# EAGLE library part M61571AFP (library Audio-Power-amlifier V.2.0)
M61571AFP is a Digital power amplifier IC developed for home audio. M61571AFP can realize maximum Power 50W × 2ch(VD = 21V,THD = 10%, BTL) at 4 Ω load. It is possible to replace from the conventional analog amplifier system to the digital amplifier system easily. Refer to "http://www.renesas.com/en/network" for the latest and detailed information.
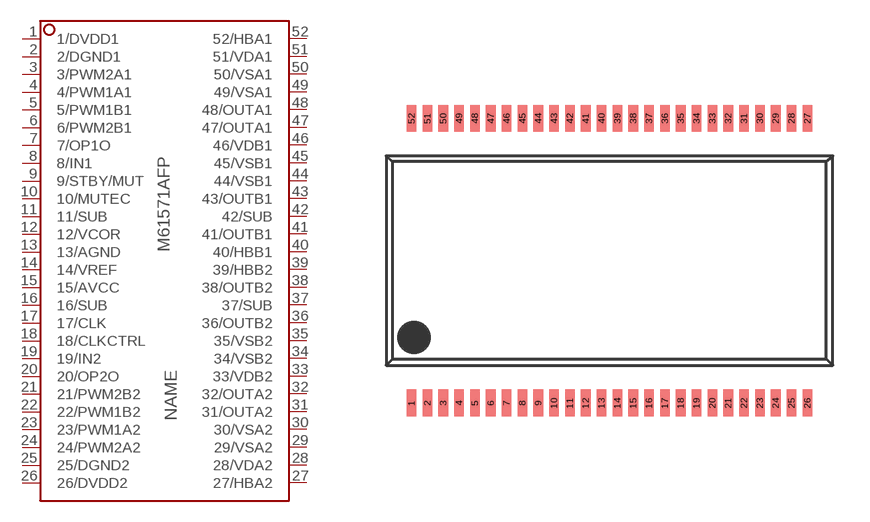
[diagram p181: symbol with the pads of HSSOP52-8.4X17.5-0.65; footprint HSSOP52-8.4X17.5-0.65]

Designator prefix IC

## M61571AFP  [HSSOP52-8.4X17.5-0.65]
1  1/DVDD1  pwr
2  2/DGND1  pwr
3  3/PWM2A1
4  4/PWM1A1
5  5/PWM1B1
6  6/PWM2B1
7  7/OP1O  out
8  8/IN1  in
9  9/STBY/MUT  in
10  10/MUTEC  in
11  11/SUB
12  12/VCOR
13  13/AGND  pwr
14  14/VREF  pwr
15  15/AVCC  pwr
16  16/SUB
17  17/CLK
18  18/CLKCTRL
19  19/IN2  in
20  20/OP2O  out
21  21/PWM2B2
22  22/PWM1B2
23  23/PWM1A2
24  24/PWM2A2
25  25/DGND2  pwr
26  26/DVDD2  pwr
27  27/HBA2
28  28/VDA2  pwr
29  29/VSA2  out
30  30/VSA2  out
31  31/OUTA2  out
32  32/OUTA2  out
33  33/VDB2  pwr
34  34/VSB2  pwr
35  35/VSB2  pwr
36  36/OUTB2  pwr
37  37/SUB
38  38/OUTB2  out
39  39/HBB2
40  40/HBB1
41  41/OUTB1  out
42  42/SUB
43  43/OUTB1  out
44  44/VSB1  out
45  45/VSB1  out
46  46/VDB1  out
47  47/OUTA1  out
48  48/OUTA1  out
49  49/VSA1  out
50  50/VSA1  out
51  51/VDA1  out
52  52/HBA1

## Footprint HSSOP52-8.4X17.5-0.65 (pad centres in mm)
P-HSSOP52-8.4x17.5-0.65
smd 0.4 x 1.1: 1 -7.8,-5.85; 2 -7.15,-5.85; 3 -6.5,-5.85; 4 -5.85,-5.85; 5 -5.2,-5.85; 6 -4.55,-5.85; 7 -3.9,-5.85; 8 -3.25,-5.85; 9 -2.6,-5.85; 10 -1.95,-5.85; 11 -1.3,-5.85; 12 -0.65,-5.85; 13 0,-5.85; 14 0.65,-5.85; 15 1.3,-5.85; 16 1.95,-5.85; 17 2.6,-5.85; 18 3.25,-5.85; 19 3.9,-5.85; 20 4.55,-5.85; 21 5.2,-5.85; 22 5.85,-5.85; 23 6.5,-5.85; 24 7.15,-5.85; 25 7.8,-5.85; 26 8.45,-5.85; 27 8.45,5.85; 28 7.8,5.85; 29 7.15,5.85; 30 6.5,5.85; 31 5.85,5.85; 32 5.2,5.85; 33 4.55,5.85; 34 3.9,5.85; 35 3.25,5.85; 36 2.6,5.85; 37 1.95,5.85; 38 1.3,5.85; 39 0.65,5.85; 40 0,5.85; 41 -0.65,5.85; 42 -1.3,5.85; 43 -1.95,5.85; 44 -2.6,5.85; 45 -3.25,5.85; 46 -3.9,5.85; 47 -4.55,5.85; 48 -5.2,5.85; 49 -5.85,5.85; 50 -6.5,5.85; 51 -7.15,5.85; 52 -7.8,5.85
